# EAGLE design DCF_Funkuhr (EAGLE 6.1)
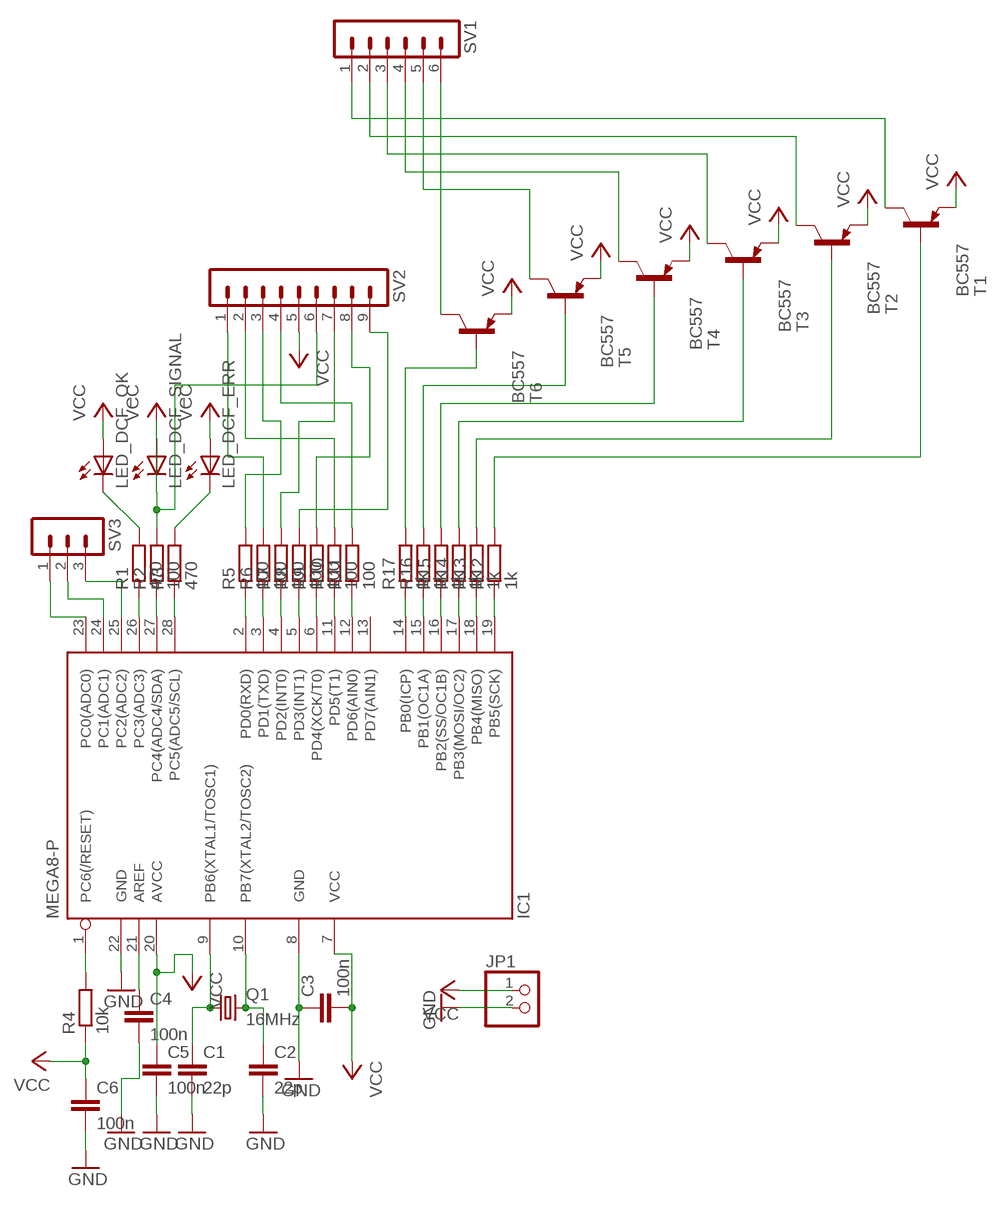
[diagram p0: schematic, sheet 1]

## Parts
C1  22p  C-EU050-024X044  [C050-024X044]
C2  22p  C-EU050-024X044  [C050-024X044]
C3  100n  C-EU050-025X075  [C050-025X075]
C4  100n  C-EU050-025X075  [C050-025X075]
C5  100n  C-EU050-025X075  [C050-025X075]
C6  100n  C-EU050-025X075  [C050-025X075]
IC1  MEGA8-P  [DIL28-3]
JP1  PINHD-1X2  [1X02]
LED_DCF_ERR  LED3MM  [LED3MM]
LED_DCF_OK  LED3MM  [LED3MM]
LED_DCF_SIGNAL  LED3MM  [LED3MM]
Q1  16MHz  CRYSTALHC49S  [HC49/S]
R1  470  R-EU_0207/10  [0207/10]
R2  100  R-EU_0207/10  [0207/10]
R3  470  R-EU_0207/10  [0207/10]
R4  10k  R-EU_0207/10  [0207/10]
R5  100  R-EU_0207/10  [0207/10]
R6  100  R-EU_0207/10  [0207/10]
R7  100  R-EU_0207/10  [0207/10]
R8  100  R-EU_0207/10  [0207/10]
R9  100  R-EU_0207/10  [0207/10]
R10  100  R-EU_0207/10  [0207/10]
R11  100  R-EU_0207/10  [0207/10]
R12  1k  R-EU_0207/10  [0207/10]
R13  1k  R-EU_0207/10  [0207/10]
R14  1k  R-EU_0207/10  [0207/10]
R15  1k  R-EU_0207/10  [0207/10]
R16  1k  R-EU_0207/10  [0207/10]
R17  1k  R-EU_0207/10  [0207/10]
SV1  MA06-1  [MA06-1]
SV2  MA09-1  [MA09-1]
SV3  MA03-1  [MA03-1]
T1  BC557  [TO92-EBC]
T2  BC557  [TO92-EBC]
T3  BC557  [TO92-EBC]
T4  BC557  [TO92-EBC]
T5  BC557  [TO92-EBC]
T6  BC557  [TO92-EBC]

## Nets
GND: C1.2 C2.2 C3.1 C4.2 C5.2 C6.2 IC1.8(GND) IC1.22(GND) JP1.2
N$1: R17.2 T6.B
N$2: R16.2 T5.B
N$3: R15.2 T4.B
N$4: R14.2 T3.B
N$5: R13.2 T2.B
N$6: R12.2 T1.B
N$7: SV1.6 T6.C
N$8: SV1.5 T5.C
N$9: SV1.4 T4.C
N$10: SV1.3 T3.C
N$11: SV1.2 T2.C
N$12: SV1.1 T1.C
N$13: IC1.14(PB0(ICP)) R17.1
N$14: IC1.15(PB1(OC1A)) R16.1
N$15: IC1.16(PB2(SS/OC1B)) R15.1
N$16: IC1.17(PB3(MOSI/OC2)) R14.1
N$17: IC1.18(PB4(MISO)) R13.1
N$18: IC1.19(PB5(SCK)) R12.1
N$19: LED_DCF_OK.K(C) R1.2
N$21: LED_DCF_ERR.K(C) R3.2
N$22: C4.1 IC1.21(AREF)
N$23: IC1.23(PC0(ADC0)) SV3.1
N$24: C1.1 IC1.9(PB6(XTAL1/TOSC1)) Q1.1
N$25: C2.1 IC1.10(PB7(XTAL2/TOSC2)) Q1.2
N$26: IC1.1(PC6(/RESET)) R4.2
N$27: LED_DCF_SIGNAL.K(C) R2.2 SV2.6
N$28: IC1.12(PD6(AIN0)) R11.1
N$29: IC1.11(PD5(T1)) R10.1
N$30: IC1.6(PD4(XCK/T0)) R9.1
N$31: IC1.5(PD3(INT1)) R8.1
N$32: IC1.4(PD2(INT0)) R7.1
N$33: IC1.3(PD1(TXD)) R6.1
N$34: IC1.2(PD0(RXD)) R5.1
N$35: IC1.28(PC5(ADC5/SCL)) R3.1
N$36: IC1.27(PC4(ADC4/SDA)) R2.1
N$37: IC1.26(PC3(ADC3)) R1.1
N$38: R6.2 SV2.1
N$39: R10.2 SV2.2
N$40: R5.2 SV2.3
N$41: R11.2 SV2.4
N$42: R7.2 SV2.7
N$43: R9.2 SV2.8
N$44: R8.2 SV2.9
N$45: IC1.24(PC1(ADC1)) SV3.2
N$46: IC1.25(PC2(ADC2)) SV3.3
VCC: C3.2 C5.1 C6.1 IC1.7(VCC) IC1.20(AVCC) JP1.1 LED_DCF_ERR.A LED_DCF_OK.A LED_DCF_SIGNAL.A R4.1 SV2.5 T1.E T2.E T3.E T4.E T5.E T6.E
Unconnected: IC1.13(PD7(AIN1))

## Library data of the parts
C1-C6 = rcl:C-EU: CAPACITOR, European symbol
IC1 = atmel:MEGA8-P: MICROCONTROLLER 8 Kbytes FLASH, 1 kbytes SRAM, 512 bytes EEPROM, USART, 4-channel 10 bit ADC, 2-channel 8 bit ADC Pin compatible with Atmega48, ATMega88, ATMega168 Source: avr.lbr; OC_FARNELL: unknown; OC_NEWARK: unknown
JP1 = pinhead:PINHD-1X2: PIN HEADER
LED_DCF_ERR LED_DCF_OK LED_DCF_SIGNAL = led:LED: LED
Q1 = crystal:CRYSTAL: CRYSTAL; OC_FARNELL: 1667008; OC_NEWARK: unknown
R1-R17 = rcl:R-EU_: RESISTOR, European symbol
SV1 = con-lstb:MA06-1: PIN HEADER
SV2 = con-lstb:MA09-1: PIN HEADER
SV3 = con-lstb:MA03-1: PIN HEADER; OC_FARNELL: unknown; OC_NEWARK: unknown
T1-T6 = transistor-pnp:BC557*: PNP Transistror

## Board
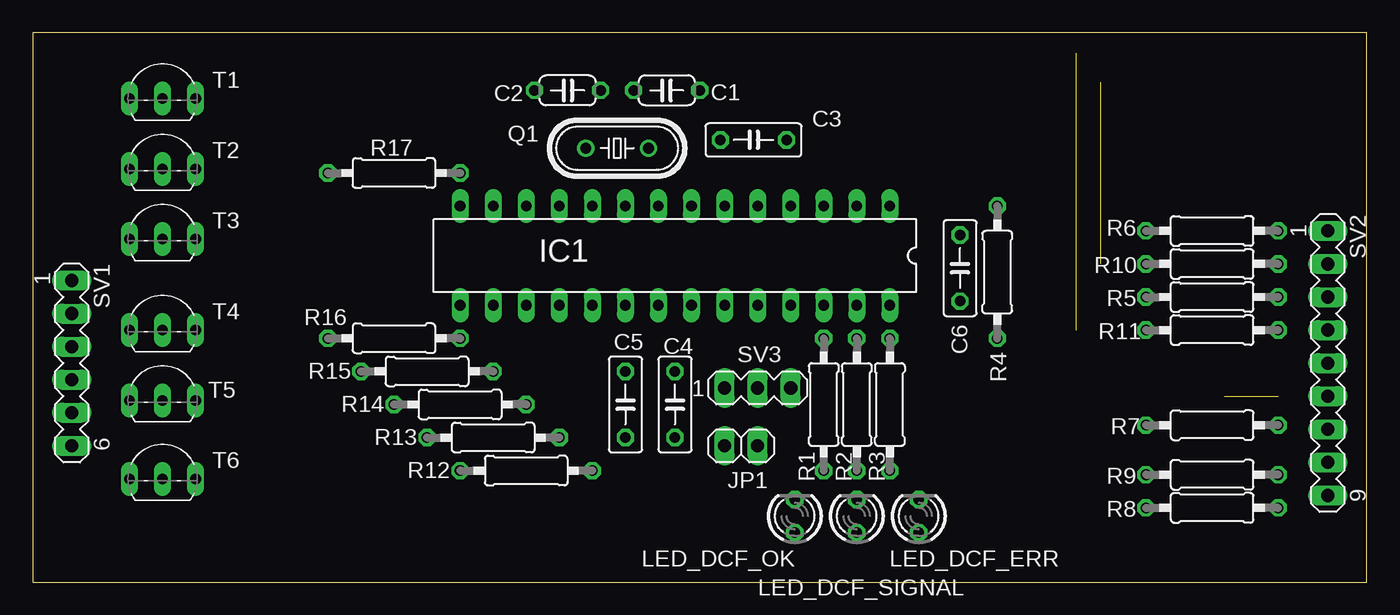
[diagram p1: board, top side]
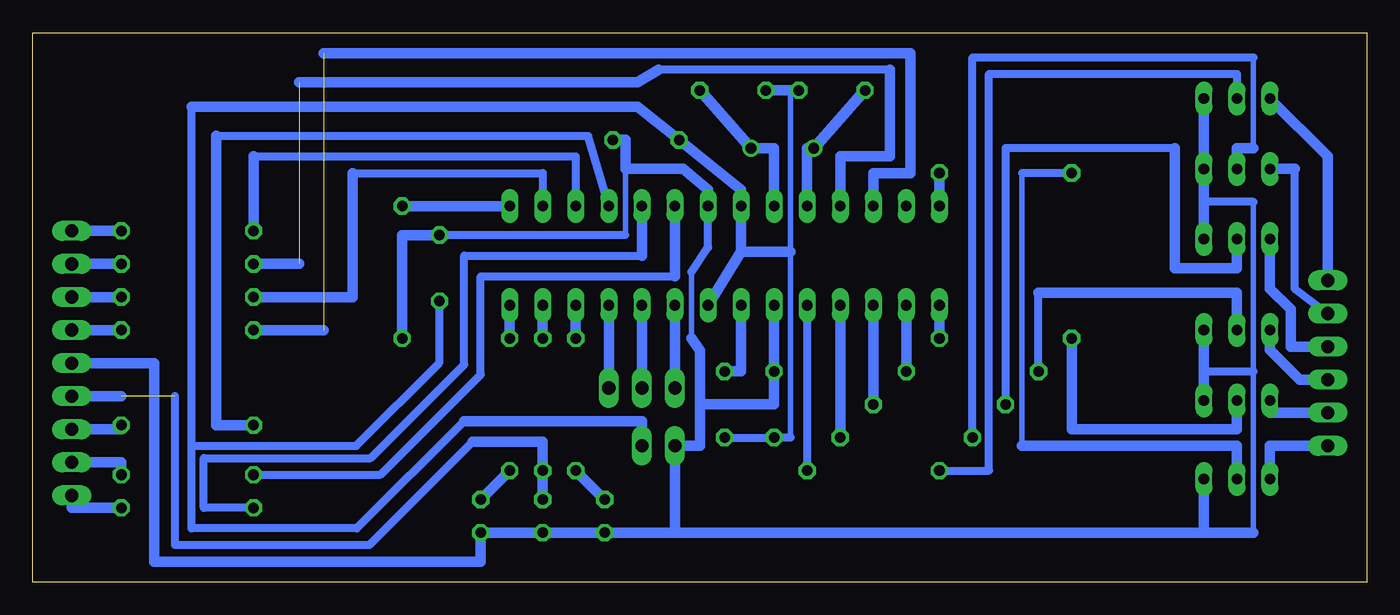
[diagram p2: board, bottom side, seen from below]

Size 102.54 x 42.22 mm. Coordinates in mm from the lower left corner, seen from the top.
Outline: 0,0 102.54,0 102.54,42.22 0,42.22 0,0
Copper layers 1*16: Top 0.035mm / dielectric 1.5mm / Bottom 0.035mm
Design rules: minimum track width 16mil, minimum drill 24mil, track to track 10mil, track to pad 10mil, pad to pad 8mil, via to via 8mil, smd to smd 8mil, copper to edge 40mil, drill to drill 8mil, minimum pad ring 10mil, minimum via ring 8mil, stop-mask expansion 4mil, vias tented up to drill 0mil, thermal gap 10mil

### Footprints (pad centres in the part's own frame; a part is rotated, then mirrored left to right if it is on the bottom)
C050-024X044 = drill 0.813 octagon: 1 -2.54,0; 2 2.54,0
C050-025X075 = drill 0.813 octagon: 1 -2.54,0; 2 2.54,0
DIL28-3 = drill 0.813 long: 1 -16.51,-3.81; 2 -13.97,-3.81; 3 -11.43,-3.81; 4 -8.89,-3.81; 5 -6.35,-3.81; 6 -3.81,-3.81; 7 -1.27,-3.81; 8 1.27,-3.81; 9 3.81,-3.81; 10 6.35,-3.81; 11 8.89,-3.81; 12 11.43,-3.81; 13 13.97,-3.81; 14 16.51,-3.81; 15 16.51,3.81; 16 13.97,3.81; 17 11.43,3.81; 18 8.89,3.81; 19 6.35,3.81; 20 3.81,3.81; 21 1.27,3.81; 22 -1.27,3.81; 23 -3.81,3.81; 24 -6.35,3.81; 25 -8.89,3.81; 26 -11.43,3.81; 27 -13.97,3.81; 28 -16.51,3.81
1X02 = drill 1.016 long: 1 -1.27,0; 2 1.27,0
LED3MM = drill 0.813 octagon: A -1.27,0; K 1.27,0
HC49/S = drill 0.813: 1 -2.413,0; 2 2.413,0
0207/10 = drill 0.813 octagon: 1 -5.08,0; 2 5.08,0
MA06-1 = drill 1.016 long: 1 -6.35,0; 2 -3.81,0; 3 -1.27,0; 4 1.27,0; 5 3.81,0; 6 6.35,0
MA09-1 = drill 1.016 long: 1 -10.16,0; 2 -7.62,0; 3 -5.08,0; 4 -2.54,0; 5 0,0; 6 2.54,0; 7 5.08,0; 8 7.62,0; 9 10.16,0
MA03-1 = drill 1.016 long: 1 -2.54,0; 2 0,0; 3 2.54,0
TO92-EBC = drill 0.813 long: B 0,-1.27; C -2.54,-1.27; E 2.54,-1.27

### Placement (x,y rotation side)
C1  48.73,37.78 180 top
C2  41.11,37.78 0 top
C3  55.4,33.97 0 top
C4  49.36,13.65 270 top
C5  45.55,13.65 270 top
C6  71.27,24.12 270 top
IC1  49.36,25.08 180 top
JP1  54.45,10.47 0 top
LED_DCF_ERR  68.1,5.08 90 top
LED_DCF_OK  58.57,5.08 90 top
LED_DCF_SIGNAL  63.33,5.08 90 top
Q1  44.92,33.33 180 top
R1  60.79,13.65 270 top
R2  63.33,13.65 270 top
R3  65.88,13.65 270 top
R4  74.13,23.81 90 top
R5  90.64,21.9 0 top
R6  90.64,26.98 0 top
R7  90.64,12.06 0 top
R8  90.64,5.71 0 top
R9  90.64,8.25 0 top
R10  90.64,24.44 0 top
R11  90.64,19.36 0 top
R12  37.93,8.57 180 top
R13  35.39,11.11 180 top
R14  32.85,13.65 180 top
R15  30.32,16.19 180 top
R16  27.78,18.73 180 top
R17  27.78,31.43 180 top
SV1  3.01,16.82 270 top
SV2  99.53,16.82 270 top
SV3  55.71,14.92 0 top
T1  10,38.41 0 top
T2  10,33.02 0 top
T3  10,27.62 0 top
T4  10,20.63 0 top
T5  10,15.23 0 top
T6  10,9.2 0 top

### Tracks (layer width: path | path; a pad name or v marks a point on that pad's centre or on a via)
GND
  Bottom 0.406: 44.28,37.78 44.28,25.39 44.28,11.11 | C5.2 46.51,11.11
  Bottom 0.61: C4.2 C5.2 44.28,11.11 | 90.32,10.47 90.32,36.51 | 90.32,10.47 77.66,10.47 71.27,16.86 C6.2 | 69.37,12.38 77.62,4.12 90.32,4.12 90.32,10.47
  Bottom 0.813: C1.2 44.28,37.78 C2.2 | 48.09,25.39 IC1.22 | 48.09,25.39 IC1.8 48.09,30.16 C3.1 56.03,36.51 90.32,36.51 | 48.09,25.39 44.28,25.39 | JP1.2 55.71,12.38 69.37,12.38
N$1
  Bottom 0.406: 26.5,31.43 26.5,10.47
  Bottom 0.61: R17.2 26.5,31.43
  Bottom 0.813: 26.5,10.47 10,10.47 T6.B
N$2
  Bottom 0.813: T5.B 10,11.74 22.7,11.74 R16.2
N$3
  Bottom 0.61: R15.2 25.23,22.22
  Bottom 0.813: T4.B 10,22.22 25.23,22.22
N$4
  Bottom 0.61: R14.2 27.78,33.33 14.76,33.33
  Bottom 0.813: 14.76,33.33 14.76,24.12 10,24.12 T3.B
N$5
  Bottom 0.406: 8.72,40.32 8.72,33.33
  Bottom 0.61: 8.72,40.32 30.32,40.32 R13.2
  Bottom 0.813: T2.B 10,33.33 8.72,33.33
N$6
  Bottom 0.61: T1.B 10,39.05 29.05,39.05 29.05,8.57 R12.2
N$7
  Bottom 0.813: SV1.6 7.46,10.47 T6.C
N$8
  Bottom 0.813: T5.C 7.46,13.01 SV1.5
N$9
  Bottom 0.813: SV1.4 5.16,15.55 7.46,17.84 T4.C
N$10
  Bottom 0.813: T3.C 7.46,22.54 5.87,20.95 5.87,18.09 SV1.3
N$11
  Bottom 0.61: 5.55,31.75 5.55,22.54 SV1.2
  Bottom 0.813: 5.55,31.75 T2.C
N$12
  Bottom 0.813: T1.C 3.01,32.7 SV1.1
N$13
  Bottom 0.813: R17.1 IC1.14
N$14
  Bottom 0.813: IC1.15 R16.1
N$15
  Bottom 0.813: IC1.16 R15.1
N$16
  Bottom 0.813: IC1.17 R14.1
N$17
  Bottom 0.813: IC1.18 R13.1
N$18
  Bottom 0.61: IC1.19 R12.1
N$19
  Bottom 0.813: LED_DCF_OK.K R1.2
N$21
  Bottom 0.813: R3.2 LED_DCF_ERR.K
N$22
  Bottom 0.813: C4.1 48.09,16.19 IC1.21
N$23
  Bottom 0.813: SV3.1 IC1.23
N$24
  Bottom 0.813: IC1.9 45.55,33.33 Q1.1 C1.1
N$25
  Bottom 0.406: 43.01,33.33 Q1.2
  Bottom 0.813: 43.01,33.33 IC1.10 | Q1.2 C2.1
N$26
  Bottom 0.813: IC1.1 R4.2
N$27  (1 unrouted)
  Bottom 0.61: 91.59,14.28 91.59,2.85 76.67,2.85 68.73,10.79
  Bottom 0.813: LED_DCF_SIGNAL.K R2.2 63.33,10.79 68.73,10.79 | SV2.6 95.72,14.28
N$28  (1 unrouted)
  Bottom 0.813: IC1.12 37.93,31.43 35.08,31.43 35.08,40.63 80.16,40.63 | R11.1 80.16,19.36
N$29  (1 unrouted)
  Bottom 0.61: 36.66,39.37 54.45,39.37
  Bottom 0.813: IC1.11 40.47,32.7 36.66,32.7 36.66,39.37 | 82.07,38.41 56.03,38.41 54.45,39.37 | R10.1 82.07,24.44
N$30
  Bottom 0.61: 53.17,23.49 68.1,23.49 68.1,15.95 75.79,8.25 R9.1
  Bottom 0.813: 53.17,23.49 IC1.6
N$31
  Bottom 0.61: R8.1 89.37,5.71 89.37,9.52 76.57,9.52 69.37,16.72 69.37,25.08 55.71,25.08
  Bottom 0.813: 55.71,25.08 IC1.5
N$32
  Bottom 0.61: 88.42,34.28 59.84,34.28 IC1.4
  Bottom 0.813: 88.42,34.28 88.42,12.06 R7.1
N$33
  Bottom 0.61: IC1.3 60.79,32.7 85.56,32.7
  Bottom 0.813: R6.1 85.56,32.7
N$34
  Bottom 0.61: IC1.2 63.33,31.43 77.94,31.43
  Bottom 0.813: 77.94,31.43 77.94,21.9 R5.1
N$35
  Bottom 0.813: IC1.28 R3.1
N$36
  Bottom 0.813: IC1.27 R2.1
N$37
  Bottom 0.813: IC1.26 R1.1
N$38
  Bottom 0.813: SV2.1 R6.2
N$39
  Bottom 0.813: SV2.2 R10.2
N$40
  Bottom 0.813: SV2.3 R5.2
N$41
  Bottom 0.813: SV2.4 R11.2
N$42
  Bottom 0.61: 95.72,11.74 R7.2
  Bottom 0.813: SV2.7 95.72,11.74
N$43
  Bottom 0.813: SV2.8 95.72,9.2 R9.2
N$44
  Bottom 0.813: SV2.9 99.53,5.71 R8.2
N$45
  Bottom 0.813: SV3.2 IC1.24
N$46
  Bottom 0.813: SV3.3 IC1.25
VCC
  Bottom 0.406: 8.72,3.81 8.72,16.19 8.72,29.2 | 51.9,18.73 51.9,23.81 | 56.98,26.66 56.98,31.75
  Bottom 0.61: 12.54,16.19 8.72,16.19 | 8.72,29.2 12.54,29.2 | 56.98,26.66 C6.1 | 51.9,23.81 50.63,25.71 IC1.7
  Bottom 0.813: T1.E T2.E 12.54,29.2 T3.E | 8.72,3.81 12.54,3.81 | T5.E 12.54,16.19 T4.E | IC1.7 50.63,30.16 52.54,31.75 56.98,31.75 56.98,33.97 C3.2 | IC1.20 C5.1 45.55,13.65 51.27,13.65 | 53.17,3.81 JP1.1 51.27,10.47 51.27,13.65 | 51.27,13.65 51.27,17.77 51.9,18.73 | 12.54,3.81 T6.E | 53.17,3.81 12.54,3.81 | 53.17,3.81 LED_DCF_OK.A LED_DCF_SIGNAL.A LED_DCF_ERR.A 68.1,1.58 93.18,1.58 93.18,16.82 SV2.5 | C6.1 74.13,26.66 R4.1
